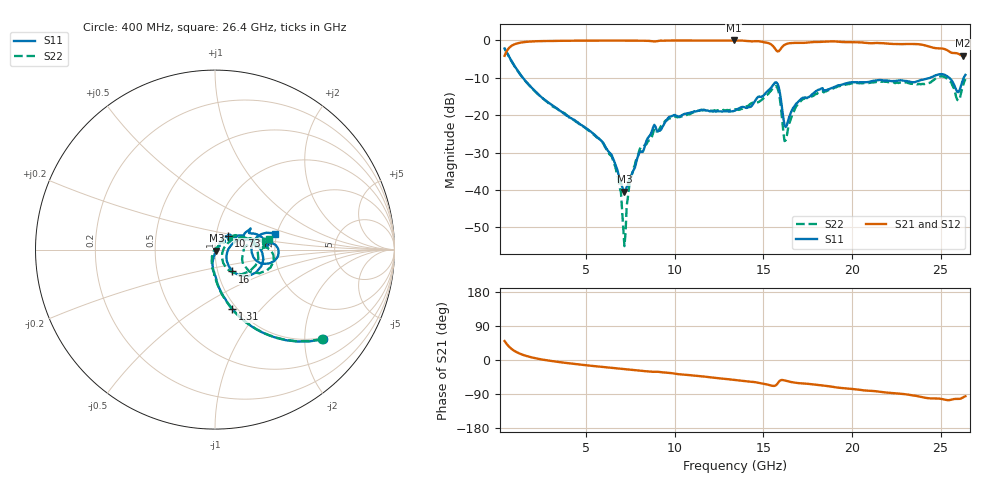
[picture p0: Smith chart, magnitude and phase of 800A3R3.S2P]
!  American Technical Ceramics  Date:  9/12/2007
!  One Norden Lane
!  Huntington Station,  NY.  11746-2102
!  Tel:  (631) 622-4700  Fax:  (631) 622-4748
!  Part Number  800A3R3  Mounting Orientation: Vertical
!  Description: Ultra Low ESR Microwave capacitors
!  Application: Coupling, Bypass, Tuning, DC Block
!  Filters, Matching
# GHZ S DB R 50
! Freq  |S11|  S11 Ph  |S21|  S21 Ph  |S12|  S12 Ph  |S22|  S22 Ph
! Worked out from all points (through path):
!   401 points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, 400 MHz to 26.4 GHz, reference 50 ohm
!   highest |S21| = 0.00 dB at 13.34 GHz (marker M1); lowest = -4.1 dB at 26.27 GHz (marker M2)
!   group delay of S21, straight-line fit = 12.7 ps
!   lowest |S11| = -40.4 dB at 7.16 GHz (marker M3), VSWR 1.02, Z = 50.8 - j0.581 ohm
!   |S11| at or under -10 dB: 1.435 GHz to 24.4 GHz (22.97 GHz wide, 178 % of centre); 25.49 GHz to 26.31 GHz (817.9 MHz wide, 3.16 % of centre)
!   |S22| runs from -55.0 to -2.2 dB; largest |S21 - S12| = 0.013
!   S11 on the Smith chart (normalised r, x): 400 MHz: 0.95, -2.44; 1.31 GHz: 0.95, -0.72; 10.73 GHz: 1.14, +0.18; 16 GHz: 1.18, -0.29; 26.4 GHz: 1.96, +0.38
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0.4  -2.14 -39.8  -4.10 49.9  -4.14 49.9  -2.19 -40.0
1.31  -9.24 -73.8  -0.57 15.8  -0.61 15.8  -9.29 -74.0
4.755  -22.69 -100.5  -0.05 -12.6  -0.07 -12.4  -22.78 -103.5
6.51  -31.51 -94.0  -0.02 -21.1  -0.01 -20.9  -31.99 -117.1
6.835  -36.05 -81.4  -0.03 -22.7  -0.02 -22.4  -37.73 -124.4
7.16  -40.43 -37.0  -0.05 -24.2  -0.03 -23.9  -55.04 160.5
7.55  -36.19 15.1  -0.06 -25.9  -0.04 -25.6  -36.41 45.8
7.94  -30.88 39.8  -0.06 -27.6  -0.04 -27.3  -30.54 46.5
9.11  -24.19 44.4  -0.10 -31.3  -0.06 -31.0  -23.83 46.1
10.735  -19.44 47.3  -0.01 -39.5  -0.01 -39.5  -19.80 35.4
13.335  -18.86 35.6  0.00 -52.5  -0.01 -52.6  -18.49 35.9
13.4  -18.77 35.6  -0.02 -52.8  -0.01 -52.9  -18.43 35.8
15.675  -11.21 -11.2  -2.28 -67.5  -2.24 -67.9  -12.16 -11.8
16  -16.13 -51.4  -2.11 -53.0  -2.08 -53.2  -18.31 -59.2
16.26  -23.17 -13.5  -1.02 -54.7  -0.98 -54.9  -26.72 -1.4
16.91  -16.69 22.7  -0.66 -60.7  -0.61 -60.9  -17.28 27.2
17.755  -14.38 29.0  -0.45 -64.2  -0.40 -64.5  -14.93 18.7
22.11  -10.78 3.8  -0.88 -86.7  -0.85 -87.3  -11.11 6.7
25.62  -10.65 -15.6  -3.29 -104.6  -3.27 -105.3  -11.45 -29.0
26.01  -13.82 4.2  -3.58 -102.8  -3.58 -103.6  -16.10 -6.9
26.27  -10.42 18.2  -4.11 -98.8  -4.09 -99.7  -12.05 14.4
26.4  -9.22 14.3  -3.98 -95.7  -3.97 -96.5  -10.35 10.9
